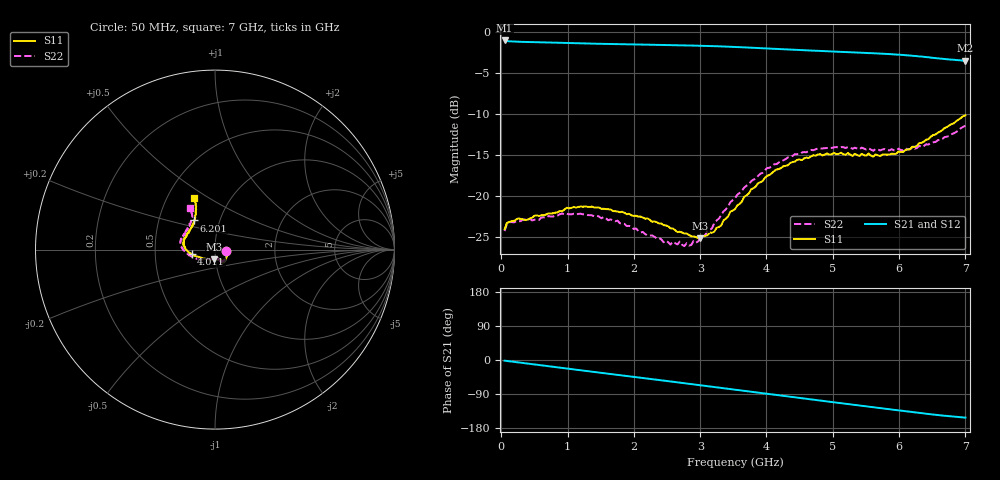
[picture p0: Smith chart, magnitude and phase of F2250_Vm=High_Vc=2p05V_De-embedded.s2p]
! Integrated Device Technology
! Corporate Headquarters
! 6024 Silver Creek Valley Road
! San Jose, CA 95138  USA
! Phone:  1-408-284-8200
! Toll Free:  1-800-223-1366
! Webpage:  http://www.idt.com/
! Timing and RF Division
! 515 Groton Road, Suite 102
! Westford, MA 01886-6024
! Device:  F2250
! Description: Voltage Variable RF Attenuator
! Frequency:  50.0 -  6000.00 MHz
! Package:  3x3 mm Thin QFN Plastic Package: 16 pin
! Ports:  2 RF, 3 DC
!  Pin  1  = GND
!  Pin  2  = NC
!  Pin  3  = RF1  = Port 1
!  Pin  4  = NC
!  Pin  5  = GND
!  Pin  6  = GND
!  Pin  7  = GND
!  Pin  8  = GND
!  Pin  9  = NC
!  Pin 10  = RF2  = Port 2
!  Pin 11  = NC
!  Pin 12  = GND
!  Pin 13  = GND
!  Pin 14  = VCNTRL
!  Pin 15  = VDD
!  Pin 16  = VMODE
! Vcntrl:  2.050 Volts
! Vmode:  +3.300 Volts
! Vdd:  +3.30  Volts
! Current:  1.318 mA
! Data:  The device was measured on a the F2250 evaluation board which has
!  individual transmission lines to the RF pins.  Data was collected
!  using a calibrated network analyzer.  The evaluation board was
!  de-embedded using a TRL calibration technique.
!  The reference plane is the edge of the package pin.
! Misc:  SN 10
!  Action Tracker AT0258
! Date Measured:  2014-11-26
! Date:  2015-10-15  MJV
! Note:
!  Integrated Device Technology supplies this data as a sample of measured
!  data at the package pin for this product.  Your particular data for this
!  product may vary.
!  Data was taken at 25 degrees C.
!  Integrated Device Technology reserves the right to change this data at anytime.
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# GHz S dB R 50
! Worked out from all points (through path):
!   201 points, 50 MHz to 7 GHz, reference 50 ohm
!   highest |S21| = -0.99 dB at 50 MHz (marker M1); lowest = -3.5 dB at 7 GHz (marker M2)
!   group delay of S21, straight-line fit = 61.1 ps
!   lowest |S11| = -25.2 dB at 3.004 GHz (marker M3), VSWR 1.12, Z = 49.2 - j5.41 ohm
!   |S11| at or under -10 dB: start of sweep to end of sweep
!   |S22| runs from -26.2 to -11.4 dB; largest |S21 - S12| = 0.0019
!   S11 on the Smith chart (normalised r, x): 50 MHz: 1.13, -0.02; 4.011 GHz: 0.77, -0.04; 6.201 GHz: 0.75, +0.26; 7 GHz: 0.68, +0.43
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0.05  -24.09 -9.0  -0.99 -1.8  -0.99 -1.8  -24.31 -9.6
0.1195  -23.21 -8.9  -1.09 -3.3  -1.09 -3.2  -23.22 -8.1
0.91875  -21.89 -45.2  -1.28 -21.0  -1.28 -21.1  -22.15 -48.2
1.2315  -21.34 -53.0  -1.35 -27.9  -1.35 -27.9  -22.26 -58.6
1.75275  -21.91 -59.8  -1.44 -39.1  -1.44 -39.1  -23.03 -66.2
2.37825  -23.38 -60.3  -1.53 -52.7  -1.53 -52.8  -25.15 -69.2
2.552  -23.97 -64.7  -1.56 -56.6  -1.56 -56.6  -25.97 -75.8
2.691  -24.39 -71.5  -1.58 -59.7  -1.58 -59.7  -25.60 -82.9
2.7605  -24.61 -73.4  -1.59 -61.3  -1.59 -61.3  -26.16 -87.1
2.93425  -25.03 -87.1  -1.63 -65.1  -1.63 -65.2  -25.74 -101.8
3.00375  -25.18 -95.6  -1.64 -66.7  -1.64 -66.7  -25.08 -109.1
3.21225  -24.39 -117.6  -1.69 -71.4  -1.69 -71.4  -23.35 -127.7
3.525  -21.64 -145.1  -1.79 -78.5  -1.79 -78.5  -20.28 -146.4
3.76825  -19.20 -159.3  -1.88 -84.0  -1.88 -84.0  -18.21 -157.8
4.0115  -17.55 -168.6  -1.97 -89.4  -1.97 -89.4  -16.59 -167.4
4.4285  -15.81 179.5  -2.13 -98.6  -2.14 -98.6  -14.91 179.9
4.7065  -15.03 172.2  -2.23 -104.8  -2.24 -104.8  -14.42 174.0
5.054  -14.89 164.0  -2.36 -112.4  -2.36 -112.5  -14.03 166.8
5.85325  -14.94 137.7  -2.66 -129.9  -2.66 -130.0  -14.44 147.8
6.20075  -13.98 125.7  -2.87 -137.6  -2.87 -137.7  -14.05 138.7
6.54825  -12.50 117.3  -3.14 -144.7  -3.14 -144.8  -13.41 127.3
7  -10.15 112.1  -3.47 -152.0  -3.48 -152.1  -11.43 121.0
